| TEXAS INSTRUMENTS INCORPORATED
| Clock Distribution Circuits
| IBIS Model of SSTUB32866
| 25-Bit Configurable Registered DDR2 DIMM Buffer
| This file contains package information for the following:
| LFBGA 96-pin (ZKE) package as [Component] SN74SSTUB32866_11A for the 1:1 Reg
| LFBGA 96-pin (ZKE) package as [Component] SN74SSTUB32866_12A for the 1:2 RegA
| LFBGA 96-pin (ZKE) package as [Component] SN74SSTUB32866_12B for the 1:2 RegB
[IBIS Ver]   4.0
[File name]   sstub32866_zke1.ibs
[File Rev]   1.1
[Date]   Jun 29 11:38:59 MEST 2007
[Source]   From Texas Instruments LVCMOS HSPICE models
[Notes]   File created by SIEMENS AG / I&S IT SCS MCH 4
   An IBIS model does not adequately simulate the dynamic
   behavior of the multi-stage output driver in the SN74SSTU32864
   device. TI recommends that customers do NOT use the IBIS model.
   For more accurate simulation results, please use the HSPICE
   model if you can.
   Rev. 1.1: weak model of the Output_buffer_Q866 improved
[Disclaimer]   Data is for modeling purposes only and is not guaranteed.
|   IBIS Open Forum disclaims all warranties. See DISCLAIM.TXT in
|   vhdl.org:/pub/IBIS/models for the full disclaimer.
[Copyright]   (C) Copyright  by SIEMENS AG / I&S IT SCS MCH 4
| Component: SN74SSTUB32866_11A Package  LFBGA-ZKE
[Component]   SN74SSTUB32866_11A
[Manufacturer]   Texas_Instruments
[Package]
|   typ   min   max
R_pkg   77.1m   1.0m   117.0m
L_pkg   2.28nH   0.219nH   3.47nH
C_pkg   0.199pF   0.061pF   0.281pF
[Pin]   signal_name   model_name   R_pin   L_pin   C_pin
A3   VREF1   Input_buffer_Ddiv3   8.20E-02  2.54E-09  1.96E-13
B3   GND   GND   6.60E-02  1.83E-09  1.67E-13
A2   PPO   Output_buffer_PPO   9.10E-02  2.73E-09  1.97E-13
A1   DCKE   Input_buffer_Ddiv3   1.09E-01  3.06E-09  2.31E-13
B2   D15   Input_buffer_Ddiv3   1.08E-01  2.97E-09  2.47E-13
B1   D2   Input_buffer_Ddiv3   1.03E-01  2.87E-09  2.36E-13
C3   VCC   POWER   2.00E-02  1.07E-09  1.17E-13
C2   D16   Input_buffer_Ddiv3   9.50E-02  2.67E-09  2.23E-13
C1   D3   Input_buffer_Ddiv3   8.80E-02  2.44E-09  2.15E-13
D3   GND   GND   1.02E-01  3.11E-09  2.63E-13
D2   QERR   Output_buffer_QERR   8.20E-02  2.35E-09  2.13E-13
D1   DODT   Input_buffer_Ddiv3   7.70E-02  2.18E-09  1.97E-13
E3   VCC   POWER   9.40E-02  2.93E-09  2.52E-13
E2   D17   Input_buffer_Ddiv3   7.20E-02  2.10E-09  1.95E-13
E1   D5   Input_buffer_Ddiv3   6.80E-02  1.94E-09  1.80E-13
F3   GND   GND   8.20E-02  2.58E-09  2.23E-13
F2   D18   Input_buffer_Ddiv3   6.00E-02  1.74E-09  1.65E-13
F1   D6   Input_buffer_Ddiv3   5.90E-02  1.73E-09  1.68E-13
G3   VCC   POWER   7.50E-02  2.43E-09  2.17E-13
G2   NRESET  Input_buffer_LVCMOS   5.40E-02  1.58E-09  1.56E-13
G1   PAR_IN  Input_buffer_D1x   5.40E-02  1.58E-09  1.60E-13
H3   GND   GND   6.90E-02  2.25E-09  2.01E-13
H2   DCS   Input_buffer_D2x   5.00E-02  1.53E-09  1.48E-13
H1   CLK   Input_buffer_CLK   5.20E-02  1.62E-09  1.53E-13
J1   NCLK   Input_buffer_CLK   5.30E-02  1.63E-09  1.49E-13
J2   CSR   Input_buffer_D2x   6.00E-03  4.22E-10  7.40E-14
J3   VCC   POWER   6.90E-02  2.25E-09  1.98E-13
K1   D8   Input_buffer_Ddiv3   5.40E-02  1.58E-09  1.60E-13
K2   D19   Input_buffer_Ddiv3   5.40E-02  1.58E-09  1.56E-13
K3   GND   GND   7.50E-02  2.43E-09  2.17E-13
L1   D9   Input_buffer_Ddiv3   5.90E-02  1.73E-09  1.68E-13
L2   D20   Input_buffer_Ddiv3   6.00E-02  1.74E-09  1.65E-13
L3   VCC   POWER   8.20E-02  2.58E-09  2.23E-13
M1   D10   Input_buffer_Ddiv3   6.80E-02  1.94E-09  1.80E-13
M2   D21   Input_buffer_Ddiv3   7.20E-02  2.10E-09  1.95E-13
M3   GND   GND   9.40E-02  2.93E-09  2.52E-13
N1   D11   Input_buffer_Ddiv3   7.70E-02  2.18E-09  1.97E-13
N2   D22   Input_buffer_Ddiv3   8.20E-02  2.35E-09  2.13E-13
N3   VCC   POWER   1.02E-01  3.11E-09  2.63E-13
P1   D12   Input_buffer_Ddiv3   8.80E-02  2.44E-09  2.15E-13
P2   D23   Input_buffer_Ddiv3   9.50E-02  2.67E-09  2.23E-13
P3   GND   GND   2.00E-02  1.07E-09  1.17E-13
R1   D13   Input_buffer_Ddiv3   1.03E-01  2.87E-09  2.36E-13
R2   D24   Input_buffer_Ddiv3   1.08E-01  2.97E-09  2.47E-13
T1   D14   Input_buffer_Ddiv3   1.09E-01  3.06E-09  2.31E-13
T2   D25   Input_buffer_Ddiv3   9.10E-02  2.73E-09  1.87E-13
R3   VCC   POWER   1.00E-03  2.19E-10  6.10E-14
T3   VREF48  Input_buffer_Ddiv3   8.20E-02  2.54E-09  1.96E-13
T4   VCC   POWER   8.20E-02  2.54E-09  2.10E-13
R4   VCC   POWER   6.60E-02  1.83E-09  1.67E-13
T5   Q14   Output_buffer_Q866   9.10E-02  2.73E-09  1.92E-13
T6   Q25   Output_buffer_Q866   1.09E-01  3.06E-09  2.30E-13
R5   Q13   Output_buffer_Q866   1.08E-01  2.96E-09  2.45E-13
R6   Q24   Output_buffer_Q866   1.03E-01  2.85E-09  2.42E-13
P4   GND   GND   1.17E-01  3.47E-09  2.81E-13
P5   Q12   Output_buffer_Q866   9.90E-02  2.77E-09  2.36E-13
P6   Q23   Output_buffer_Q866   9.20E-02  2.54E-09  2.24E-13
N4   VCC   POWER   1.05E-01  3.18E-09  2.69E-13
N5   Q11   Output_buffer_Q866   8.50E-02  2.43E-09  2.16E-13
N6   Q22   Output_buffer_Q866   8.00E-02  2.26E-09  2.01E-13
M4   GND   GND   9.70E-02  3.00E-09  2.55E-13
M5   Q10   Output_buffer_Q866   7.50E-02  2.17E-09  1.98E-13
M6   Q21   Output_buffer_Q866   7.10E-02  2.01E-09  1.85E-13
L4   VCC   POWER   8.40E-02  2.62E-09  2.24E-13
L5   Q9   Output_buffer_Q866   6.20E-02  1.79E-09  1.69E-13
L6   Q20   Output_buffer_Q866   6.00E-02  1.75E-09  1.71E-13
K4   GND   GND   7.60E-02  2.44E-09  2.16E-13
K5   Q8   Output_buffer_Q866   5.40E-02  1.59E-09  1.56E-13
K6   Q19   Output_buffer_Q866   5.50E-02  1.59E-09  1.59E-13
J4   VCC   POWER   6.90E-02  2.26E-09  2.00E-13
J5   NC   NC   5.00E-02  1.53E-09  1.49E-13
J6   NC   NC   5.20E-02  1.62E-09  1.60E-13
H6   DNU   NC   5.20E-02  1.62E-09  1.60E-13
H5   QCS   Output_buffer_Q866   5.00E-02  1.53E-09  1.49E-13
H4   GND   GND   6.90E-02  2.26E-09  2.00E-13
G6   C0   Input_buffer_LVCMOS   5.50E-02  1.59E-09  1.59E-13
G5   C1   Input_buffer_LVCMOS   5.40E-02  1.59E-09  1.56E-13
G4   VCC   POWER   7.60E-02  2.44E-09  2.17E-13
F6   Q18   Output_buffer_Q866   6.00E-02  1.75E-09  1.71E-13
F5   Q6   Output_buffer_Q866   6.20E-02  1.79E-09  1.69E-13
F4   GND   GND   8.40E-02  2.62E-09  2.24E-13
E6   Q17   Output_buffer_Q866   7.10E-02  2.01E-09  1.85E-13
E5   Q5   Output_buffer_Q866   7.50E-02  2.17E-09  1.98E-13
E4   VCC   POWER   9.70E-02  3.00E-09  2.55E-13
D6   DNU   NC   8.00E-02  2.26E-09  2.01E-13
D5   QODT   Output_buffer_Q866   8.50E-02  2.43E-09  2.16E-13
D4   GND   GND   1.05E-01  3.18E-09  2.69E-13
C6   Q16   Output_buffer_Q866   9.20E-02  2.54E-09  2.24E-13
C5   Q3   Output_buffer_Q866   9.90E-02  2.77E-09  2.36E-13
C4   VCC   POWER   1.17E-01  3.47E-09  2.81E-13
B6   Q15   Output_buffer_Q866   1.03E-01  2.85E-09  2.42E-13
B5   Q2   Output_buffer_Q866   1.08E-01  2.96E-09  2.45E-13
A6   DNU   NC   1.09E-01  3.06E-09  2.30E-13
A5   QCKE   Output_buffer_Q866   9.10E-02  2.73E-09  1.95E-13
B4   GND   GND   6.60E-02  1.83E-09  1.69E-13
A4   VCC   POWER   8.20E-02  2.54E-09  2.00E-13
|********************** DIFF PIN **********************************************
[Diff_pin]   inv_pin   vdiff   tdelay_typ   tdelay_min   tdelay_max
   H1   J1   .350V   0ns   NA   NA
| Component: SN74SSTUB32866_12A Package  LFBGA-ZKE
[Component]   SN74SSTUB32866_12A
[Manufacturer]   Texas_Instruments
[Package]
|   typ   min   max
R_pkg   77.1m   1.0m   117.0m
L_pkg   2.28nH   0.219nH   3.47nH
C_pkg   0.199pF   0.061pF   0.281pF
[Pin]   signal_name   model_name   R_pin   L_pin   C_pin
A3   VREF1   Input_buffer_Ddiv3   8.20E-02  2.54E-09  1.96E-13
B3   GND   GND   6.60E-02  1.83E-09  1.67E-13
A2   PPO   Output_buffer_PPO   9.10E-02  2.73E-09  1.97E-13
A1   DCKE   Input_buffer_Ddiv3   1.09E-01  3.06E-09  2.31E-13
B2   DNU   NC   1.08E-01  2.97E-09  2.47E-13
B1   D2   Input_buffer_Ddiv3   1.03E-01  2.87E-09  2.36E-13
C3   VCC   POWER   2.00E-02  1.07E-09  1.17E-13
C2   DNU   NC   9.50E-02  2.67E-09  2.23E-13
C1   D3   Input_buffer_Ddiv3   8.80E-02  2.44E-09  2.15E-13
D3   GND   GND   1.02E-01  3.11E-09  2.63E-13
D2   QERR   Output_buffer_QERR   8.20E-02  2.35E-09  2.13E-13
D1   DODT   Input_buffer_Ddiv3   7.70E-02  2.18E-09  1.97E-13
E3   VCC   POWER   9.40E-02  2.93E-09  2.52E-13
E2   DNU   NC   7.20E-02  2.10E-09  1.95E-13
E1   D5   Input_buffer_Ddiv3   6.80E-02  1.94E-09  1.80E-13
F3   GND   GND   8.20E-02  2.58E-09  2.23E-13
F2   DNU   NC   6.00E-02  1.74E-09  1.65E-13
F1   D6   Input_buffer_Ddiv3   5.90E-02  1.73E-09  1.68E-13
G3   VCC   POWER   7.50E-02  2.43E-09  2.17E-13
G2   NRESET  Input_buffer_LVCMOS   5.40E-02  1.58E-09  1.56E-13
G1   PAR_IN  Input_buffer_D1x   5.40E-02  1.58E-09  1.60E-13
H3   GND   GND   6.90E-02  2.25E-09  2.01E-13
H2   DCS   Input_buffer_D2x   5.00E-02  1.53E-09  1.48E-13
H1   CLK   Input_buffer_CLK   5.20E-02  1.62E-09  1.53E-13
J1   NCLK   Input_buffer_CLK   5.30E-02  1.63E-09  1.49E-13
J2   CSR   Input_buffer_D2x   6.00E-03  4.22E-10  7.40E-14
J3   VCC   POWER   6.90E-02  2.25E-09  1.98E-13
K1   D8   Input_buffer_Ddiv3   5.40E-02  1.58E-09  1.60E-13
K2   DNU   NC   5.40E-02  1.58E-09  1.56E-13
K3   GND   GND   7.50E-02  2.43E-09  2.17E-13
L1   D9   Input_buffer_Ddiv3   5.90E-02  1.73E-09  1.68E-13
L2   DNU   NC   6.00E-02  1.74E-09  1.65E-13
L3   VCC   POWER   8.20E-02  2.58E-09  2.23E-13
M1   D10   Input_buffer_Ddiv3   6.80E-02  1.94E-09  1.80E-13
M2   DNU   NC   7.20E-02  2.10E-09  1.95E-13
M3   GND   GND   9.40E-02  2.93E-09  2.52E-13
N1   D11   Input_buffer_Ddiv3   7.70E-02  2.18E-09  1.97E-13
N2   DNU   NC   8.20E-02  2.35E-09  2.13E-13
N3   VCC   POWER   1.02E-01  3.11E-09  2.63E-13
P1   D12   Input_buffer_Ddiv3   8.80E-02  2.44E-09  2.15E-13
P2   DNU   NC   9.50E-02  2.67E-09  2.23E-13
P3   GND   GND   2.00E-02  1.07E-09  1.17E-13
R1   D13   Input_buffer_Ddiv3   1.03E-01  2.87E-09  2.36E-13
R2   DNU   NC   1.08E-01  2.97E-09  2.47E-13
T1   D14   Input_buffer_Ddiv3   1.09E-01  3.06E-09  2.31E-13
T2   DNU   NC   9.10E-02  2.73E-09  1.87E-13
R3   VCC   POWER   1.00E-03  2.19E-10  6.10E-14
T3   VREF48  Input_buffer_Ddiv3   8.20E-02  2.54E-09  1.96E-13
T4   VCC   POWER   8.20E-02  2.54E-09  2.10E-13
R4   VCC   POWER   6.60E-02  1.83E-09  1.67E-13
T5   Q14A   Output_buffer_Q866   9.10E-02  2.73E-09  1.92E-13
T6   Q14B   Output_buffer_Q866   1.09E-01  3.06E-09  2.30E-13
R5   Q13A   Output_buffer_Q866   1.08E-01  2.96E-09  2.45E-13
R6   Q13B   Output_buffer_Q866   1.03E-01  2.85E-09  2.42E-13
P4   GND   GND   1.17E-01  3.47E-09  2.81E-13
P5   Q12A   Output_buffer_Q866   9.90E-02  2.77E-09  2.36E-13
P6   Q12B   Output_buffer_Q866   9.20E-02  2.54E-09  2.24E-13
N4   VCC   POWER   1.05E-01  3.18E-09  2.69E-13
N5   Q11A   Output_buffer_Q866   8.50E-02  2.43E-09  2.16E-13
N6   Q11B   Output_buffer_Q866   8.00E-02  2.26E-09  2.01E-13
M4   GND   GND   9.70E-02  3.00E-09  2.55E-13
M5   Q10A   Output_buffer_Q866   7.50E-02  2.17E-09  1.98E-13
M6   Q10B   Output_buffer_Q866   7.10E-02  2.01E-09  1.85E-13
L4   VCC   POWER   8.40E-02  2.62E-09  2.24E-13
L5   Q9A   Output_buffer_Q866   6.20E-02  1.79E-09  1.69E-13
L6   Q9B   Output_buffer_Q866   6.00E-02  1.75E-09  1.71E-13
K4   GND   GND   7.60E-02  2.44E-09  2.16E-13
K5   Q8A   Output_buffer_Q866   5.40E-02  1.59E-09  1.56E-13
K6   Q8B   Output_buffer_Q866   5.50E-02  1.59E-09  1.59E-13
J4   VCC   POWER   6.90E-02  2.26E-09  2.00E-13
J5   NC   NC   5.00E-02  1.53E-09  1.49E-13
J6   NC   NC   5.20E-02  1.62E-09  1.60E-13
H6   QCSB   Output_buffer_Q866   5.20E-02  1.62E-09  1.60E-13
H5   QCSA   Output_buffer_Q866   5.00E-02  1.53E-09  1.49E-13
H4   GND   GND   6.90E-02  2.26E-09  2.00E-13
G6   C0   Input_buffer_LVCMOS   5.50E-02  1.59E-09  1.59E-13
G5   C1   Input_buffer_LVCMOS   5.40E-02  1.59E-09  1.56E-13
G4   VCC   POWER   7.60E-02  2.44E-09  2.17E-13
F6   Q6B   Output_buffer_Q866   6.00E-02  1.75E-09  1.71E-13
F5   Q6A   Output_buffer_Q866   6.20E-02  1.79E-09  1.69E-13
F4   GND   GND   8.40E-02  2.62E-09  2.24E-13
E6   Q5B   Output_buffer_Q866   7.10E-02  2.01E-09  1.85E-13
E5   Q5A   Output_buffer_Q866   7.50E-02  2.17E-09  1.98E-13
E4   VCC   POWER   9.70E-02  3.00E-09  2.55E-13
D6   QODTB   Output_buffer_Q866   8.00E-02  2.26E-09  2.01E-13
D5   QODTA   Output_buffer_Q866   8.50E-02  2.43E-09  2.16E-13
D4   GND   GND   1.05E-01  3.18E-09  2.69E-13
C6   Q3B   Output_buffer_Q866   9.20E-02  2.54E-09  2.24E-13
C5   Q3A   Output_buffer_Q866   9.90E-02  2.77E-09  2.36E-13
C4   VCC   POWER   1.17E-01  3.47E-09  2.81E-13
B6   Q2B   Output_buffer_Q866   1.03E-01  2.85E-09  2.42E-13
B5   Q2A   Output_buffer_Q866   1.08E-01  2.96E-09  2.45E-13
A6   QCKEB   Output_buffer_Q866   1.09E-01  3.06E-09  2.30E-13
A5   QCKEA   Output_buffer_Q866   9.10E-02  2.73E-09  1.95E-13
B4   GND   GND   6.60E-02  1.83E-09  1.69E-13
A4   VCC   POWER   8.20E-02  2.54E-09  2.00E-13
|********************** DIFF PIN **********************************************
[Diff_pin]   inv_pin   vdiff   tdelay_typ   tdelay_min   tdelay_max
   H1   J1   .350V   0ns   NA   NA
| Component: SN74SSTUB32866_12B Package  LFBGA-ZKE
[Component]   SN74SSTUB32866_12B
[Manufacturer]   Texas_Instruments
[Package]
|   typ   min   max
R_pkg   77.1m   1.0m   117.0m
L_pkg   2.28nH   0.219nH   3.47nH
C_pkg   0.199pF   0.061pF   0.281pF
[Pin]   signal_name   model_name   R_pin   L_pin   C_pin
A3   VREF1   Input_buffer_Ddiv3   8.20E-02  2.54E-09  1.96E-13
B3   GND   GND   6.60E-02  1.83E-09  1.67E-13
A2   PPO   Output_buffer_PPO   9.10E-02  2.73E-09  1.97E-13
A1   D1   Input_buffer_Ddiv3   1.09E-01  3.06E-09  2.31E-13
B2   DNU   NC   1.08E-01  2.97E-09  2.47E-13
B1   D2   Input_buffer_Ddiv3   1.03E-01  2.87E-09  2.36E-13
C3   VCC   POWER   2.00E-02  1.07E-09  1.17E-13
C2   DNU   NC   9.50E-02  2.67E-09  2.23E-13
C1   D3   Input_buffer_Ddiv3   8.80E-02  2.44E-09  2.15E-13
D3   GND   GND   1.02E-01  3.11E-09  2.63E-13
D2   QERR   Output_buffer_QERR   8.20E-02  2.35E-09  2.13E-13
D1   D4   Input_buffer_Ddiv3   7.70E-02  2.18E-09  1.97E-13
E3   VCC   POWER   9.40E-02  2.93E-09  2.52E-13
E2   DNU   NC   7.20E-02  2.10E-09  1.95E-13
E1   D5   Input_buffer_Ddiv3   6.80E-02  1.94E-09  1.80E-13
F3   GND   GND   8.20E-02  2.58E-09  2.23E-13
F2   DNU   NC   6.00E-02  1.74E-09  1.65E-13
F1   D6   Input_buffer_Ddiv3   5.90E-02  1.73E-09  1.68E-13
G3   VCC   POWER   7.50E-02  2.43E-09  2.17E-13
G2   NRESET  Input_buffer_LVCMOS   5.40E-02  1.58E-09  1.56E-13
G1   PAR_IN  Input_buffer_D1x   5.40E-02  1.58E-09  1.60E-13
H3   GND   GND   6.90E-02  2.25E-09  2.01E-13
H2   DCS   Input_buffer_D2x   5.00E-02  1.53E-09  1.48E-13
H1   CLK   Input_buffer_CLK   5.20E-02  1.62E-09  1.53E-13
J1   NCLK   Input_buffer_CLK   5.30E-02  1.63E-09  1.49E-13
J2   CSR   Input_buffer_D2x   6.00E-03  4.22E-10  7.40E-14
J3   VCC   POWER   6.90E-02  2.25E-09  1.98E-13
K1   D8   Input_buffer_Ddiv3   5.40E-02  1.58E-09  1.60E-13
K2   DNU   NC   5.40E-02  1.58E-09  1.56E-13
K3   GND   GND   7.50E-02  2.43E-09  2.17E-13
L1   D9   Input_buffer_Ddiv3   5.90E-02  1.73E-09  1.68E-13
L2   DNU   NC   6.00E-02  1.74E-09  1.65E-13
L3   VCC   POWER   8.20E-02  2.58E-09  2.23E-13
M1   D10   Input_buffer_Ddiv3   6.80E-02  1.94E-09  1.80E-13
M2   DNU   NC   7.20E-02  2.10E-09  1.95E-13
M3   GND   GND   9.40E-02  2.93E-09  2.52E-13
N1   DODT   Input_buffer_Ddiv3   7.70E-02  2.18E-09  1.97E-13
N2   DNU   NC   8.20E-02  2.35E-09  2.13E-13
N3   VCC   POWER   1.02E-01  3.11E-09  2.63E-13
P1   D12   Input_buffer_Ddiv3   8.80E-02  2.44E-09  2.15E-13
P2   DNU   NC   9.50E-02  2.67E-09  2.23E-13
P3   GND   GND   2.00E-02  1.07E-09  1.17E-13
R1   D13   Input_buffer_Ddiv3   1.03E-01  2.87E-09  2.36E-13
R2   DNU   NC   1.08E-01  2.97E-09  2.47E-13
T1   DCKE   Input_buffer_Ddiv3   1.09E-01  3.06E-09  2.31E-13
T2   DNU   NC   9.10E-02  2.73E-09  1.87E-13
R3   VCC   POWER   1.00E-03  2.19E-10  6.10E-14
T3   VREF48  Input_buffer_Ddiv3   8.20E-02  2.54E-09  1.96E-13
T4   VCC   POWER   8.20E-02  2.54E-09  2.10E-13
R4   VCC   POWER   6.60E-02  1.83E-09  1.67E-13
T5   QCKEA   Output_buffer_Q866   9.10E-02  2.73E-09  1.92E-13
T6   QCKEB   Output_buffer_Q866   1.09E-01  3.06E-09  2.30E-13
R5   Q13A   Output_buffer_Q866   1.08E-01  2.96E-09  2.45E-13
R6   Q13B   Output_buffer_Q866   1.03E-01  2.85E-09  2.42E-13
P4   GND   GND   1.17E-01  3.47E-09  2.81E-13
P5   Q12A   Output_buffer_Q866   9.90E-02  2.77E-09  2.36E-13
P6   Q12B   Output_buffer_Q866   9.20E-02  2.54E-09  2.24E-13
N4   VCC   POWER   1.05E-01  3.18E-09  2.69E-13
N5   QODTA   Output_buffer_Q866   8.50E-02  2.43E-09  2.16E-13
N6   QODTB   Output_buffer_Q866   8.00E-02  2.26E-09  2.01E-13
M4   GND   GND   9.70E-02  3.00E-09  2.55E-13
M5   Q10A   Output_buffer_Q866   7.50E-02  2.17E-09  1.98E-13
M6   Q10B   Output_buffer_Q866   7.10E-02  2.01E-09  1.85E-13
L4   VCC   POWER   8.40E-02  2.62E-09  2.24E-13
L5   Q9A   Output_buffer_Q866   6.20E-02  1.79E-09  1.69E-13
L6   Q9B   Output_buffer_Q866   6.00E-02  1.75E-09  1.71E-13
K4   GND   GND   7.60E-02  2.44E-09  2.16E-13
K5   Q8A   Output_buffer_Q866   5.40E-02  1.59E-09  1.56E-13
K6   Q8B   Output_buffer_Q866   5.50E-02  1.59E-09  1.59E-13
J4   VCC   POWER   6.90E-02  2.26E-09  2.00E-13
J5   NC   NC   5.00E-02  1.53E-09  1.49E-13
J6   NC   NC   5.20E-02  1.62E-09  1.60E-13
H6   QCSB   Output_buffer_Q866   5.20E-02  1.62E-09  1.60E-13
H5   QCSA   Output_buffer_Q866   5.00E-02  1.53E-09  1.49E-13
H4   GND   GND   6.90E-02  2.26E-09  2.00E-13
G6   C0   Input_buffer_LVCMOS   5.50E-02  1.59E-09  1.59E-13
G5   C1   Input_buffer_LVCMOS   5.40E-02  1.59E-09  1.56E-13
G4   VCC   POWER   7.60E-02  2.44E-09  2.17E-13
F6   Q6B   Output_buffer_Q866   6.00E-02  1.75E-09  1.71E-13
F5   Q6A   Output_buffer_Q866   6.20E-02  1.79E-09  1.69E-13
F4   GND   GND   8.40E-02  2.62E-09  2.24E-13
E6   Q5B   Output_buffer_Q866   7.10E-02  2.01E-09  1.85E-13
E5   Q5A   Output_buffer_Q866   7.50E-02  2.17E-09  1.98E-13
E4   VCC   POWER   9.70E-02  3.00E-09  2.55E-13
D6   Q4B   Output_buffer_Q866   8.00E-02  2.26E-09  2.01E-13
D5   Q4A   Output_buffer_Q866   8.50E-02  2.43E-09  2.16E-13
D4   GND   GND   1.05E-01  3.18E-09  2.69E-13
C6   Q3B   Output_buffer_Q866   9.20E-02  2.54E-09  2.24E-13
C5   Q3A   Output_buffer_Q866   9.90E-02  2.77E-09  2.36E-13
C4   VCC   POWER   1.17E-01  3.47E-09  2.81E-13
B6   Q2B   Output_buffer_Q866   1.03E-01  2.85E-09  2.42E-13
B5   Q2A   Output_buffer_Q866   1.08E-01  2.96E-09  2.45E-13
A6   Q1B   Output_buffer_Q866   1.09E-01  3.06E-09  2.30E-13
A5   Q1A   Output_buffer_Q866   9.10E-02  2.73E-09  1.95E-13
B4   GND   GND   6.60E-02  1.83E-09  1.69E-13
A4   VCC   POWER   8.20E-02  2.54E-09  2.00E-13
|********************** DIFF PIN **********************************************
[Diff_pin]   inv_pin   vdiff   tdelay_typ   tdelay_min   tdelay_max
   H1   J1   .350V   0ns   NA   NA
|   Model   Input_buffer_CLK
[Model]   Input_buffer_CLK
Model_type   Input
Polarity   Non-Inverting
Vinl   =   0.675V
Vinh   =   1.125V
|Variable   typ   min   max
C_comp   1.176e-12   9.181e-13   1.358e-12
|Variable   typ   min   max
[Voltage range]   1.8   1.7   1.9
|Variable   typ   min   max
[Temperature range]  27   125   0.0
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| Models and submodels in the file (8): Input_buffer_CLK (Input), Input_buffer_D1x (Input), Input_buffer_D2x (Input), Input_buffer_Ddiv3 (Input), Input_buffer_LVCMOS (Input), Output_buffer_PPO (Output), Output_buffer_Q866 (Output), Output_buffer_QERR (Open_drain)
